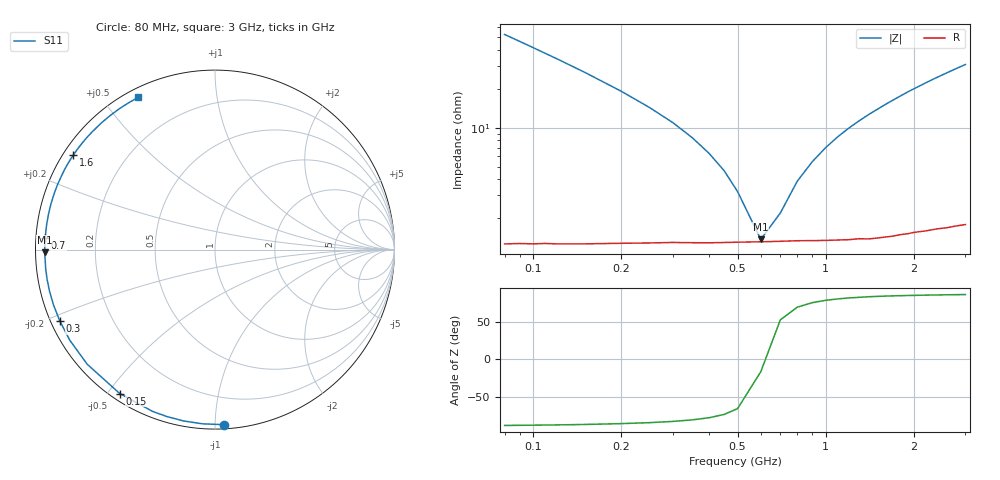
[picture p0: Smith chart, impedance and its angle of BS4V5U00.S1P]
! SIEMENS Small Signal Semiconductors
! BB640
! Si Tuning Diode in SOD323
! VR = 4.5 V
! S-Parameters:  July  1993
# GHz  S  MA  R  50
!  f  S11
! GHz  MAG  ANG
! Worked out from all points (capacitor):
!   33 points, 80 MHz to 3 GHz, reference 50 ohm
!   read as one part to ground: C = 37.1 pF near 80 MHz
!   lowest |Z| = 1.37 ohm at 600 MHz (marker M1)
!   series resonance near 618.4 MHz, so ESL is about 1.8 nH
!   S11 on the Smith chart (normalised r, x): 80 MHz: 0.03, -1.05; 150 MHz: 0.03, -0.54; 300 MHz: 0.03, -0.22; 700 MHz: 0.03, +0.03; 1.6 GHz: 0.03, +0.30; 3 GHz: 0.04, +0.62
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0.08  0.9764 -87.0
0.09  0.9732 -94.0
0.1  0.9707 -100.3
0.11  0.9681 -106.0
0.12  0.9663 -111.0
0.15  0.9616 -123.5
0.2  0.9565 -138.1
0.25  0.9537 -148.1
0.3  0.9518 -155.4
0.35  0.9511 -161.2
0.4  0.9506 -165.9
0.45  0.95 -169.8
0.5  0.9495 -173.3
0.6  0.949 -179.1
0.7  0.9486 176.0
0.8  0.9483 171.7
0.9  0.9485 167.9
1  0.9487 164.3
1.2  0.949 157.7
1.4  0.9495 151.8
1.6  0.9491 146.4
1.8  0.9484 141.3
2  0.948 136.5
2.2  0.9483 132.0
2.4  0.9482 127.8
2.6  0.9489 123.9
2.8  0.9491 120.2
3  0.9497 116.7
